(* Logix 5000 AddOnInstructionDefinition export PRNG; software revision 30.00; part 2 of 3 *)

ADD_ON_INSTRUCTION L_ADD   (* revision 1.0 00 Release, vendor Rockwell Automation *)
// Add (64-bit)
// Revision note:
// Initial Release
// Help:
// Adds two LINT (signed 64-bit) values and returns a LINT (signed 64-bit) sum.
// Also provides math status bits for Carry, Negative, Overflow and Zero result
// (equivalent to built-in S:C, S:N, S:V, S:Z).
VAR_IN_OUT
   Inp_A : LINT; {required}   // First Addend, 64-bit Integer
   Inp_B : LINT; {required}   // Second Addend, 64-bit Integer
   Out : LINT; {required}   // Sum, 64-bit Integer
END_VAR
VAR_OUTPUT
   Sts_C : BOOL; {access Read Only, visible}   // Carry result
   Sts_N : BOOL; {access Read Only, visible}   // Negative result
   Sts_V : BOOL; {access Read Only, visible}   // Overflow result
   Sts_Z : BOOL; {access Read Only, visible}   // Zero result
END_VAR
VAR
   Wrk_Sum : DINT[3];   // 20- and 24-bit fields of Out (sum)
   Wrk_B : DINT[3];   // 20- and 24-bit fields of Inp_B
   Wrk_A : DINT[3];   // 20- and 24-bit fields of Inp_A
   Wrk_Out : DINT[2];   // Output as two 32-bit DINTs
   Wrk_InpB : DINT[2];   // Input B as two 32-bit DINTs
   Wrk_InpA : DINT[2];   // Input A as two 32-bit DINTs
END_VAR

ROUTINE Logic   (* ladder *)
// Do 64-bit addition
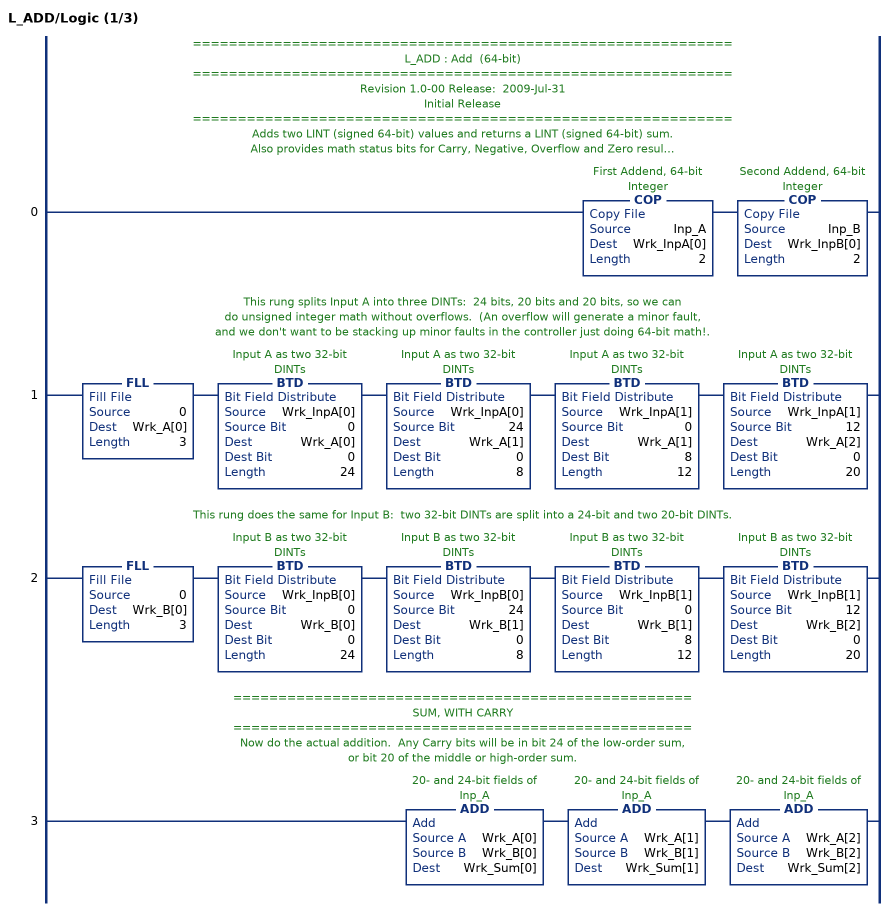
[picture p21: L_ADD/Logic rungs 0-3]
   // ============================================================
   // L_ADD : Add  (64-bit)
   // ============================================================
   // Revision 1.0-00 Release:  2009-Jul-31
   // Initial Release
   // ============================================================
   // Adds two LINT (signed 64-bit) values and returns a LINT (signed 64-bit) sum.
   // Also provides math status bits for Carry, Negative, Overflow and Zero result
   // (equivalent to built-in S:C, S:N, S:V, S:Z).
   // This instruction breaks the LINT addends into three DINTs
   // (24 bits, 20 bits and 20 bits) to do the math in order to
   // avoid generating a Controller MINOR FAULT on overflow.
   // (Sample code provided in RSLogix 5000 Online Help is much
   // smaller and faster, but causes numerous Minor Faults on
   // Overflows -- S:V -- on the low-order sum!  The controller must
   // take time to log the minor faults, and many users do not want to see
   // Minor Faults on normal math operations.  See the RSLogix 5000
   // Help Topic "Arithmetic Status Flags" for more information.)
   // ===================================================
   // CONVERT LINTs TO DINTs
   // ===================================================
   // These COPies take the input LINTs and break them into pairs of DINTs so we can do math on them.
   // Logix V17 has a LINT data type, but math instructions (and AOI Input and Output Parameters) don't support LINT.
   0: COP(Inp_A,Wrk_InpA[0],2)COP(Inp_B,Wrk_InpB[0],2);
   // This rung splits Input A into three DINTs:  24 bits, 20 bits and 20 bits, so we can
   // do unsigned integer math without overflows.  (An overflow will generate a minor fault,
   // and we don't want to be stacking up minor faults in the controller just doing 64-bit math!.
   1: FLL(0,Wrk_A[0],3)BTD(Wrk_InpA[0],0,Wrk_A[0],0,24)BTD(Wrk_InpA[0],24,Wrk_A[1],0,8)BTD(Wrk_InpA[1],0,Wrk_A[1],8,12)BTD(Wrk_InpA[1],12,Wrk_A[2],0,20);
   // This rung does the same for Input B:  two 32-bit DINTs are split into a 24-bit and two 20-bit DINTs.
   2: FLL(0,Wrk_B[0],3)BTD(Wrk_InpB[0],0,Wrk_B[0],0,24)BTD(Wrk_InpB[0],24,Wrk_B[1],0,8)BTD(Wrk_InpB[1],0,Wrk_B[1],8,12)BTD(Wrk_InpB[1],12,Wrk_B[2],0,20);
   // ===================================================
   // SUM, WITH CARRY
   // ===================================================
   // Now do the actual addition.  Any Carry bits will be in bit 24 of the low-order sum,
   // or bit 20 of the middle or high-order sum.
   3: ADD(Wrk_A[0],Wrk_B[0],Wrk_Sum[0])ADD(Wrk_A[1],Wrk_B[1],Wrk_Sum[1])ADD(Wrk_A[2],Wrk_B[2],Wrk_Sum[2]);
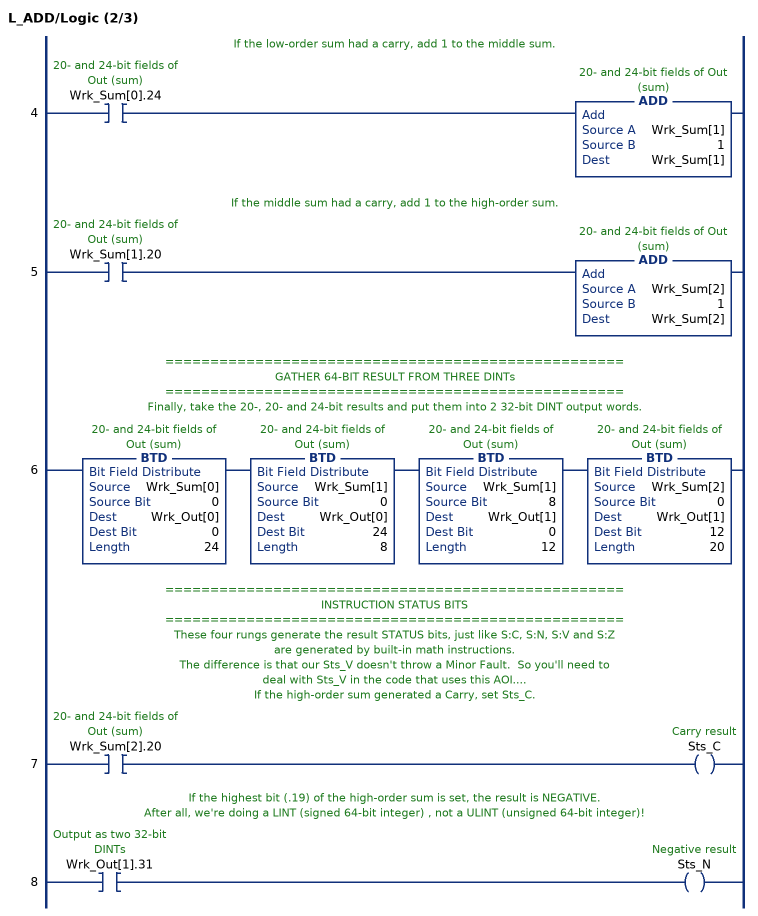
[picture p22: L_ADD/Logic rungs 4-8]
   // If the low-order sum had a carry, add 1 to the middle sum.
   4: XIC(Wrk_Sum[0].24)ADD(Wrk_Sum[1],1,Wrk_Sum[1]);
   // If the middle sum had a carry, add 1 to the high-order sum.
   5: XIC(Wrk_Sum[1].20)ADD(Wrk_Sum[2],1,Wrk_Sum[2]);
   // ===================================================
   // GATHER 64-BIT RESULT FROM THREE DINTs
   // ===================================================
   // Finally, take the 20-, 20- and 24-bit results and put them into 2 32-bit DINT output words.
   6: BTD(Wrk_Sum[0],0,Wrk_Out[0],0,24)BTD(Wrk_Sum[1],0,Wrk_Out[0],24,8)BTD(Wrk_Sum[1],8,Wrk_Out[1],0,12)BTD(Wrk_Sum[2],0,Wrk_Out[1],12,20);
   // ===================================================
   // INSTRUCTION STATUS BITS
   // ===================================================
   // These four rungs generate the result STATUS bits, just like S:C, S:N, S:V and S:Z
   // are generated by built-in math instructions.
   // The difference is that our Sts_V doesn't throw a Minor Fault.  So you'll need to
   // deal with Sts_V in the code that uses this AOI....
   // If the high-order sum generated a Carry, set Sts_C.
   7: XIC(Wrk_Sum[2].20)OTE(Sts_C);
   // If the highest bit (.19) of the high-order sum is set, the result is NEGATIVE.
   // After all, we're doing a LINT (signed 64-bit integer) , not a ULINT (unsigned 64-bit integer)!
   8: XIC(Wrk_Out[1].31)OTE(Sts_N);
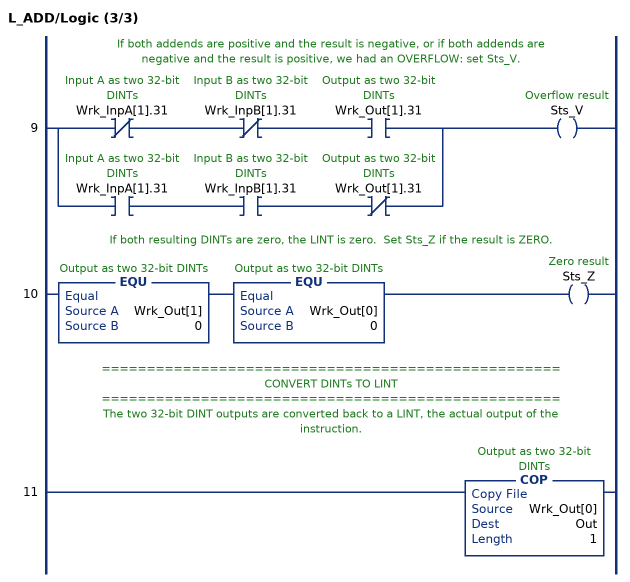
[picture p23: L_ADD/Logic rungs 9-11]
   // If both addends are positive and the result is negative, or if both addends are
   // negative and the result is positive, we had an OVERFLOW: set Sts_V.
   9: [XIO(Wrk_InpA[1].31) XIO(Wrk_InpB[1].31) XIC(Wrk_Out[1].31) ,XIC(Wrk_InpA[1].31) XIC(Wrk_InpB[1].31) XIO(Wrk_Out[1].31) ]OTE(Sts_V);
   // If both resulting DINTs are zero, the LINT is zero.  Set Sts_Z if the result is ZERO.
   10: EQU(Wrk_Out[1],0)EQU(Wrk_Out[0],0)OTE(Sts_Z);
   // ===================================================
   // CONVERT DINTs TO LINT
   // ===================================================
   // The two 32-bit DINT outputs are converted back to a LINT, the actual output of the instruction.
   11: COP(Wrk_Out[0],Out,1);
END_ROUTINE
END_ADD_ON_INSTRUCTION

ADD_ON_INSTRUCTION L_AND   (* revision 1.0 00 Release, vendor Rockwell Automation *)
// Bitwise AND (64-bit)
// Revision note:
// Initial Release
// Help:
// This instruction returns the bitwise Logical AND (output bit true if both corresponding
// input bits true) of two input 64-bit integers (LINTs), into an output 64-bit integer.
VAR_IN_OUT
   Inp_A : LINT; {required}   // Input A
   Inp_B : LINT; {required}   // Input B
   Out : LINT; {required}   // Output = Input A & Input B
END_VAR
VAR
   Wrk_Out : DINT[2];   // Output as two 32-bit DINTs
   Wrk_InpB : DINT[2];   // Input B as two 32-bit DINTs
   Wrk_InpA : DINT[2];   // Input A as two 32-bit DINTs
END_VAR

ROUTINE Logic   (* ladder *)
// Perform 64-bit bitwise logical AND
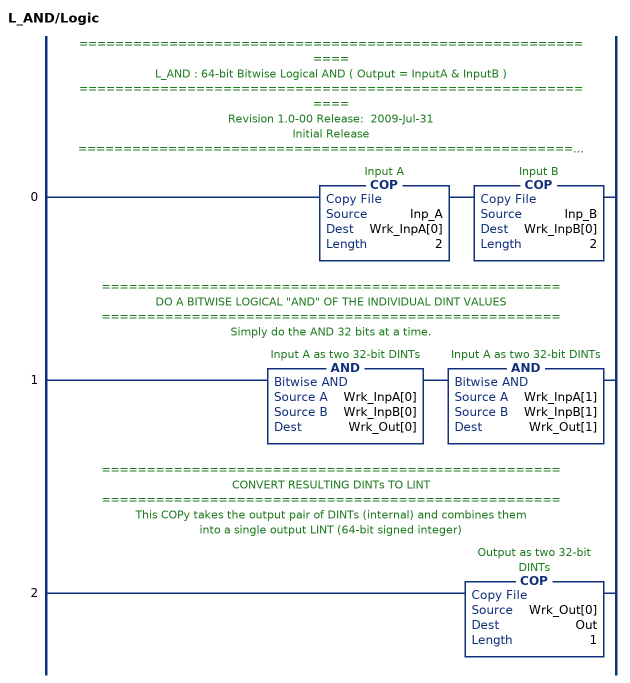
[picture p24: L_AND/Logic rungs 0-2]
   // ============================================================
   // L_AND : 64-bit Bitwise Logical AND ( Output = InputA & InputB )
   // ============================================================
   // Revision 1.0-00 Release:  2009-Jul-31
   // Initial Release
   // ============================================================
   // Returns the bitwise Logical AND of the input 64-bit integer (LINT) values.
   // This rung breaks each LINT input into two DINTs
   // (32-bit signed each) to do the logical AND function.
   // ===================================================
   // CONVERT LINTs TO DINTs
   // ===================================================
   // These COPies take the input LINT values and break them into a pair of DINTs each.
   0: COP(Inp_A,Wrk_InpA[0],2)COP(Inp_B,Wrk_InpB[0],2);
   // ===================================================
   // DO A BITWISE LOGICAL "AND" OF THE INDIVIDUAL DINT VALUES
   // ===================================================
   // Simply do the AND 32 bits at a time.
   1: AND(Wrk_InpA[0],Wrk_InpB[0],Wrk_Out[0])AND(Wrk_InpA[1],Wrk_InpB[1],Wrk_Out[1]);
   // ===================================================
   // CONVERT RESULTING DINTs TO LINT
   // ===================================================
   // This COPy takes the output pair of DINTs (internal) and combines them
   // into a single output LINT (64-bit signed integer)
   2: COP(Wrk_Out[0],Out,1);
END_ROUTINE
END_ADD_ON_INSTRUCTION

ADD_ON_INSTRUCTION L_NOT   (* revision 1.0 00 Release, vendor Rockwell Automation *)
// Bitwise NOT (64-bit)
// Revision note:
// Initial Release
// Help:
// This instruction returns the bitwise Logical NOT (inverse or 1's complement)
// of an input 64-bit integer (LINT) value.  (It flips all the bits.)
VAR_IN_OUT
   Inp : LINT; {required}   // Input
   Out : LINT; {required}   // Output = - Input
END_VAR
VAR
   Wrk : DINT[2];   // 32-bit portions of Input
END_VAR

ROUTINE Logic   (* ladder *)
// Perform a bitwise logical NOT (invert)
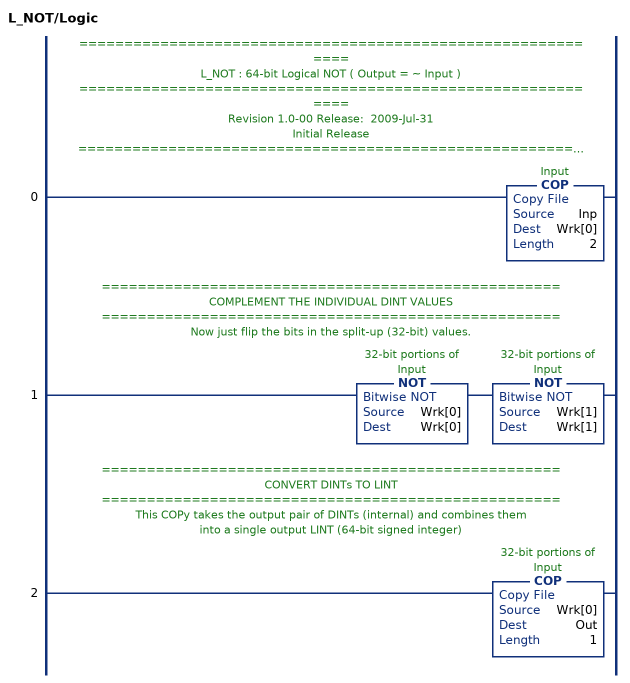
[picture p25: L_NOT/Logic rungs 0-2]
   // ============================================================
   // L_NOT : 64-bit Logical NOT ( Output = ~ Input )
   // ============================================================
   // Revision 1.0-00 Release:  2009-Jul-31
   // Initial Release
   // ============================================================
   // Returns the Logical NOT (1's complement, all bits flipped)
   // of the input 64-bit integer (LINT) value.
   // This instruction breaks the LINT input into two DINTs
   // (32-bit signed each) to do the inverting.
   // ===================================================
   // CONVERT LINT TO DINTs
   // ===================================================
   // This COPy takes the input LINT and breaks it into a pair of DINTs.
   0: COP(Inp,Wrk[0],2);
   // ===================================================
   // COMPLEMENT THE INDIVIDUAL DINT VALUES
   // ===================================================
   // Now just flip the bits in the split-up (32-bit) values.
   1: NOT(Wrk[0],Wrk[0])NOT(Wrk[1],Wrk[1]);
   // ===================================================
   // CONVERT DINTs TO LINT
   // ===================================================
   // This COPy takes the output pair of DINTs (internal) and combines them
   // into a single output LINT (64-bit signed integer)
   2: COP(Wrk[0],Out,1);
END_ROUTINE
END_ADD_ON_INSTRUCTION

ADD_ON_INSTRUCTION L_ROTR   (* revision 1.0 20170524, vendor Kenneth A. Fischer *)
// LINT circular right shift (rotation) of the 64-bit argument Inp_A by Inp_B bits
// Revision note:
// Rev1.0: 20170524 - Initial Release
VAR_IN_OUT
   Inp_A : LINT; {required}   // 64-bit Integer to be right circular rotated
END_VAR
VAR_INPUT
   Inp_B : INT; {required}   // Number of Inp_A bit rotations
END_VAR
VAR_IN_OUT
   Out : LINT; {required}   // Result
END_VAR
VAR
   Wrk_InpA : DINT[2];   // Input A as two 32-bit DINTs
   BSR_Cntrl : CONTROL := (LEN := 64);
   Source_Bit : BOOL;
   ONS : BOOL;
END_VAR

ROUTINE Logic   (* ladder *)
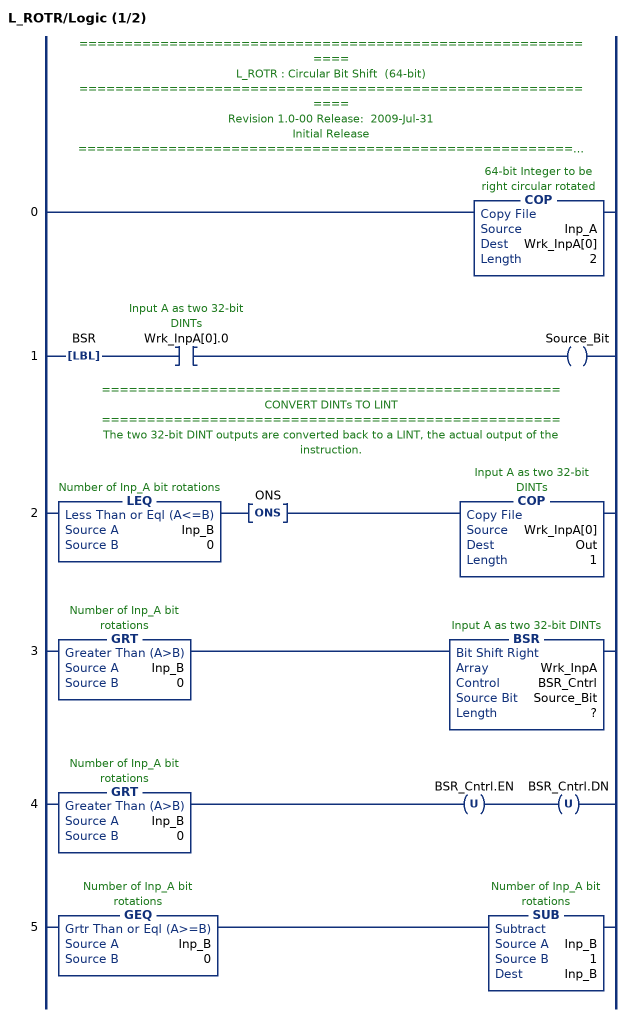
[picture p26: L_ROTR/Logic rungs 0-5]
   // ============================================================
   // L_ROTR : Circular Bit Shift  (64-bit)
   // ============================================================
   // Revision 1.0-00 Release:  2009-Jul-31
   // Initial Release
   // ============================================================
   // Performs a circular right shift rotation of the 64-bit argument Inp_A by the
   // number of bits defined in the 16-bit argument Inp_B.
   // ===================================================
   // CONVERT LINTs TO DINTs
   // ===================================================
   // These COPies take the input LINTs and break them into pairs of DINTs so we can do math on them.
   // Logix V17 has a LINT data type, but math instructions (and AOI Input and Output Parameters) don't support LINT.
   0: COP(Inp_A,Wrk_InpA[0],2);
   1: LBL(BSR)XIC(Wrk_InpA[0].0)OTE(Source_Bit);
   // ===================================================
   // CONVERT DINTs TO LINT
   // ===================================================
   // The two 32-bit DINT outputs are converted back to a LINT, the actual output of the instruction.
   2: LEQ(Inp_B,0)ONS(ONS)COP(Wrk_InpA[0],Out,1);
   3: GRT(Inp_B,0)BSR(Wrk_InpA,BSR_Cntrl,Source_Bit,?);
   4: GRT(Inp_B,0)OTU(BSR_Cntrl.EN)OTU(BSR_Cntrl.DN);
   5: GEQ(Inp_B,0)SUB(Inp_B,1,Inp_B);
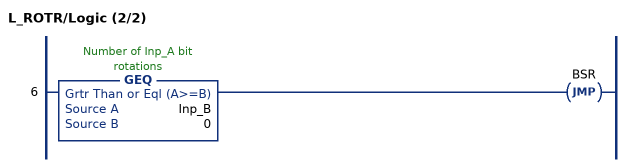
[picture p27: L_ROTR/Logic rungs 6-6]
   6: GEQ(Inp_B,0)JMP(BSR);
END_ROUTINE
END_ADD_ON_INSTRUCTION

ADD_ON_INSTRUCTION L_SHR   (* revision 1.0 20170524, vendor Kenneth A. Fischer *)
// LINT bit shift right of the 64-bit argument Inp_A by Inp_B bits with paddding by zeros on the right
// Revision note:
// Rev1.0: 20170524 - Initial Release
VAR_IN_OUT
   Inp_A : LINT; {required}   // 64-bit Integer to be right circular rotated
END_VAR
VAR_INPUT
   Inp_B : INT; {required}   // Number of bits to shift
END_VAR
VAR_IN_OUT
   Out : LINT; {required}   // Result
END_VAR
VAR
   BSR_Cntrl : CONTROL := (LEN := 64);
   ONS : BOOL;
   Source_Bit : BOOL;
   Wrk_InpA : DINT[2];   // Input A as two 32-bit DINTs
END_VAR

ROUTINE Logic   (* ladder *)
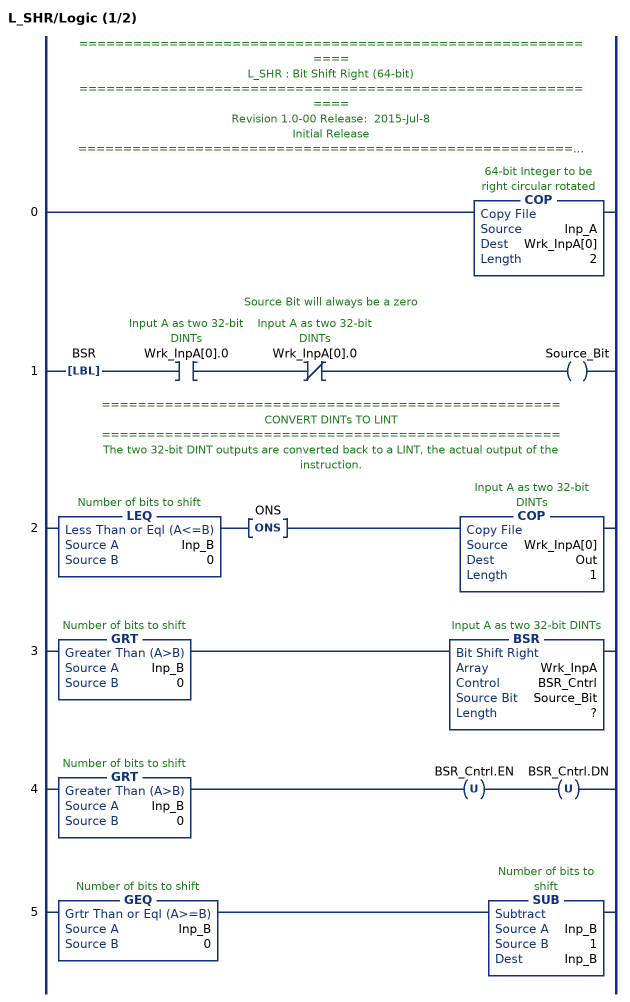
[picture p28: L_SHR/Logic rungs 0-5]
   // ============================================================
   // L_SHR : Bit Shift Right (64-bit)
   // ============================================================
   // Revision 1.0-00 Release:  2015-Jul-8
   // Initial Release
   // ============================================================
   // Performs a right bit shift of the 64-bit argument Inp_A by the
   // number of bits defined in the 16-bit argument Inp_B, with padding by zeros.
   // ===================================================
   // CONVERT LINTs TO DINTs
   // ===================================================
   // These COPies take the input LINTs and break them into pairs of DINTs so we can do math on them.
   // Logix V17 has a LINT data type, but math instructions (and AOI Input and Output Parameters) don't support LINT.
   0: COP(Inp_A,Wrk_InpA[0],2);
   // Source Bit will always be a zero
   1: LBL(BSR)XIC(Wrk_InpA[0].0)XIO(Wrk_InpA[0].0)OTE(Source_Bit);
   // ===================================================
   // CONVERT DINTs TO LINT
   // ===================================================
   // The two 32-bit DINT outputs are converted back to a LINT, the actual output of the instruction.
   2: LEQ(Inp_B,0)ONS(ONS)COP(Wrk_InpA[0],Out,1);
   3: GRT(Inp_B,0)BSR(Wrk_InpA,BSR_Cntrl,Source_Bit,?);
   4: GRT(Inp_B,0)OTU(BSR_Cntrl.EN)OTU(BSR_Cntrl.DN);
   5: GEQ(Inp_B,0)SUB(Inp_B,1,Inp_B);
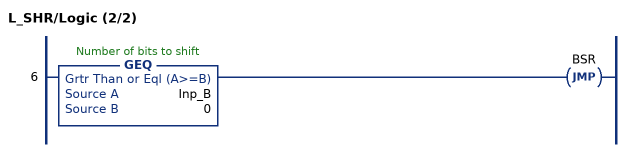
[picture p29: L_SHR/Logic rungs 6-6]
   6: GEQ(Inp_B,0)JMP(BSR);
END_ROUTINE
END_ADD_ON_INSTRUCTION

ADD_ON_INSTRUCTION L_XOR   (* revision 1.0 00 Release, vendor Rockwell Automation *)
// Bitwise XOR (64-bit)
// Revision note:
// Initial Release
// Help:
// This instruction returns the bitwise Logical XOR (exclusive OR, output
// bit true if either but NOT both of the corresponding input bits are true)
// of two input 64-bit integers (LINTs), into an output 64-bit integer.
VAR_IN_OUT
   Inp_A : LINT; {required}   // Input A
   Inp_B : LINT; {required}   // Input B
   Out : LINT; {required}   // Output = Input A | Input B
END_VAR
VAR
   Wrk_Out : DINT[2];   // Output as two 32-bit DINTs
   Wrk_InpB : DINT[2];   // Input B as two 32-bit DINTs
   Wrk_InpA : DINT[2];   // Input A as two 32-bit DINTs
END_VAR

ROUTINE Logic   (* ladder *)
// Perform bitwise logical XOR
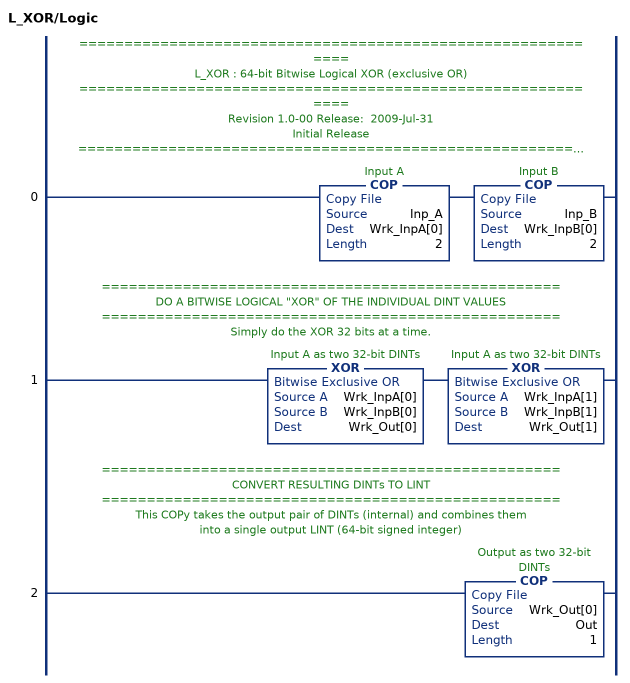
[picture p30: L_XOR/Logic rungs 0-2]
   // ============================================================
   // L_XOR : 64-bit Bitwise Logical XOR (exclusive OR)
   // ============================================================
   // Revision 1.0-00 Release:  2009-Jul-31
   // Initial Release
   // ============================================================
   // Returns the bitwise Logical XOR of the input 64-bit integer (LINT) values.
   // This rung breaks each LINT input into two DINTs
   // (32-bit signed each) to do the logical XOR function.
   // ===================================================
   // CONVERT LINTs TO DINTs
   // ===================================================
   // These COPies take the input LINT values and break them into a pair of DINTs each.
   0: COP(Inp_A,Wrk_InpA[0],2)COP(Inp_B,Wrk_InpB[0],2);
   // ===================================================
   // DO A BITWISE LOGICAL "XOR" OF THE INDIVIDUAL DINT VALUES
   // ===================================================
   // Simply do the XOR 32 bits at a time.
   1: XOR(Wrk_InpA[0],Wrk_InpB[0],Wrk_Out[0])XOR(Wrk_InpA[1],Wrk_InpB[1],Wrk_Out[1]);
   // ===================================================
   // CONVERT RESULTING DINTs TO LINT
   // ===================================================
   // This COPy takes the output pair of DINTs (internal) and combines them
   // into a single output LINT (64-bit signed integer)
   2: COP(Wrk_Out[0],Out,1);
END_ROUTINE
END_ADD_ON_INSTRUCTION

ADD_ON_INSTRUCTION SHA512_SEQ   (* revision 1.0 20170916, vendor Kenneth A. Fischer *)
// Generates SHA 512 hash of data.
// Revision note:
// Rev1.0: 20170916 - Initial Release
VAR_IN_OUT
   Inp_MSG : LINT[1600]; {required}
END_VAR
VAR_INPUT
   Inp_LEN : DINT; {required}   // LENGTH INPUT OF MSG IN NUMBER OF LINTS
END_VAR
VAR_IN_OUT
   Out_HASH : LINT[8]; {required}
        [0]   // HashBuffer_A
        [1]   // HashBuffer_B
        [2]   // HashBuffer_C
        [3]   // HashBuffer_D
        [4]   // HashBuffer_E
        [5]   // HashBuffer_F
        [6]   // HashBuffer_G
        [7]   // HashBuffer_H
END_VAR
VAR_OUTPUT
   SEQCTRL_DN : BOOL; {access Read Only}   // Complete
END_VAR
VAR_INPUT
   SEQCTRL_RESET : BOOL;   // Resets Point Multiplication if Toggled True
END_VAR
VAR_OUTPUT
   SEQCTRL_STEP : INT; {access Read Only}
END_VAR
VAR
   SEQCTRL_CMD : DINT;
   SEQCTRL_CMD_TABLE : DINT[100];
   SEQCTRL_DONE : DINT;
   SEQCTRL_NEXT_STEP : INT;
   i : INT;
   ALWAYS_OFF : BOOL;
   CondFunc : LINT;
   CondFunc_tmp : LINT[3];
   HashBuffer_A : LINT;
   HashBuffer_B : LINT;
   HashBuffer_C : LINT;
   HashBuffer_D : LINT;
   HashBuffer_E : LINT;
   HashBuffer_F : LINT;
   HashBuffer_G : LINT;
   HashBuffer_H : LINT;
   HashBufferInput_A : LINT;
   HashBufferInput_B : LINT;
   HashBufferInput_C : LINT;
   HashBufferInput_D : LINT;
   HashBufferInput_E : LINT;
   HashBufferInput_F : LINT;
   HashBufferInput_G : LINT;
   HashBufferInput_H : LINT;
   M : INT;   // MESSAGE INCREMENTS
   t : INT;
   K : LINT[85];
   L_ADD : L_ADD;
   L_ADD1 : L_ADD;
   L_AND : L_AND;
   L_NOT : L_NOT;
   L_ROTR : L_ROTR;
   L_SHR : L_SHR;
   L_XOR : L_XOR;
   LENGTH_BITS : DINT;   // LENGTH OF MSG IN BITS
   LENGTH_MODULO : DINT;
   MajFunc : LINT;
   NUM_PADDING_BITS : DINT;   // NUMBER OF BITS NEEDED FOR PADDING
   NUM_PADDING_LINTS : DINT;   // NUMBER OF LINTS NEEDED FOR PADDING
   PADDING_COUNTER : DINT;
   Sigma0 : LINT;
   Sigma1 : LINT;
   SigmaA : LINT;
   SigmaE : LINT;
   x : INT;
   j : INT;
   T1 : LINT;
   T2 : LINT;
   tmp : LINT[20];
   tmp1 : DINT;
   tmp2 : DINT;
   TOTAL_MSG_LENGTH_MINUS_16 : DINT;
   W : LINT[85];   // MESSAGE SCHEDULE
   Wrk : DINT[2];
   TEMP : DINT;
END_VAR

ROUTINE Logic   (* ladder *)
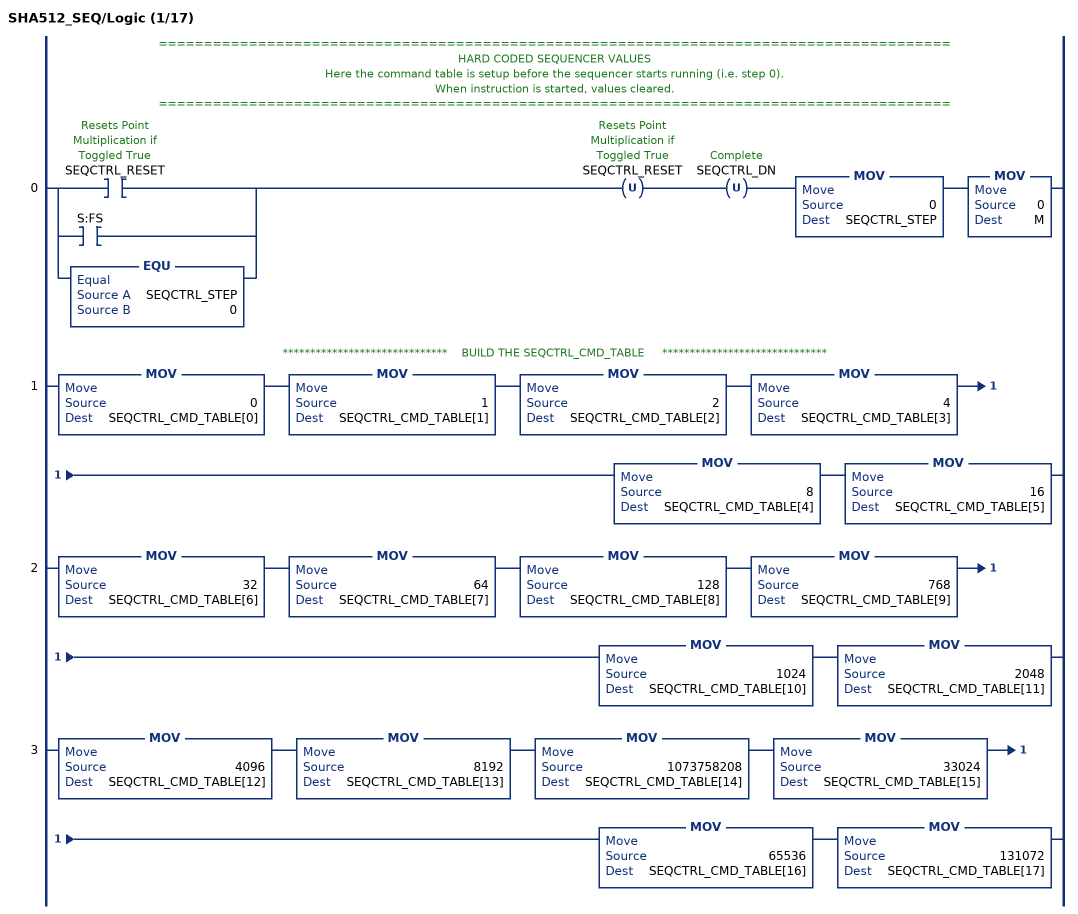
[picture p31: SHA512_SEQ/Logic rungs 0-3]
   // ========================================================================================
   // HARD CODED SEQUENCER VALUES
   // Here the command table is setup before the sequencer starts running (i.e. step 0).
   // When instruction is started, values cleared.
   // ========================================================================================
   0: [[XIC(SEQCTRL_RESET) ,XIC(S:FS) ] ,EQU(SEQCTRL_STEP,0) ]OTU(SEQCTRL_RESET)OTU(SEQCTRL_DN)MOV(0,SEQCTRL_STEP)MOV(0,M);
   // ******************************    BUILD THE SEQCTRL_CMD_TABLE     ******************************
   1: MOV(0,SEQCTRL_CMD_TABLE[0])MOV(1,SEQCTRL_CMD_TABLE[1])MOV(2,SEQCTRL_CMD_TABLE[2])MOV(4,SEQCTRL_CMD_TABLE[3])MOV(8,SEQCTRL_CMD_TABLE[4])MOV(16,SEQCTRL_CMD_TABLE[5]);
   2: MOV(32,SEQCTRL_CMD_TABLE[6])MOV(64,SEQCTRL_CMD_TABLE[7])MOV(128,SEQCTRL_CMD_TABLE[8])MOV(768,SEQCTRL_CMD_TABLE[9])MOV(1024,SEQCTRL_CMD_TABLE[10])MOV(2048,SEQCTRL_CMD_TABLE[11]);
   3: MOV(4096,SEQCTRL_CMD_TABLE[12])MOV(8192,SEQCTRL_CMD_TABLE[13])MOV(1073758208,SEQCTRL_CMD_TABLE[14])MOV(33024,SEQCTRL_CMD_TABLE[15])MOV(65536,SEQCTRL_CMD_TABLE[16])MOV(131072,SEQCTRL_CMD_TABLE[17]);
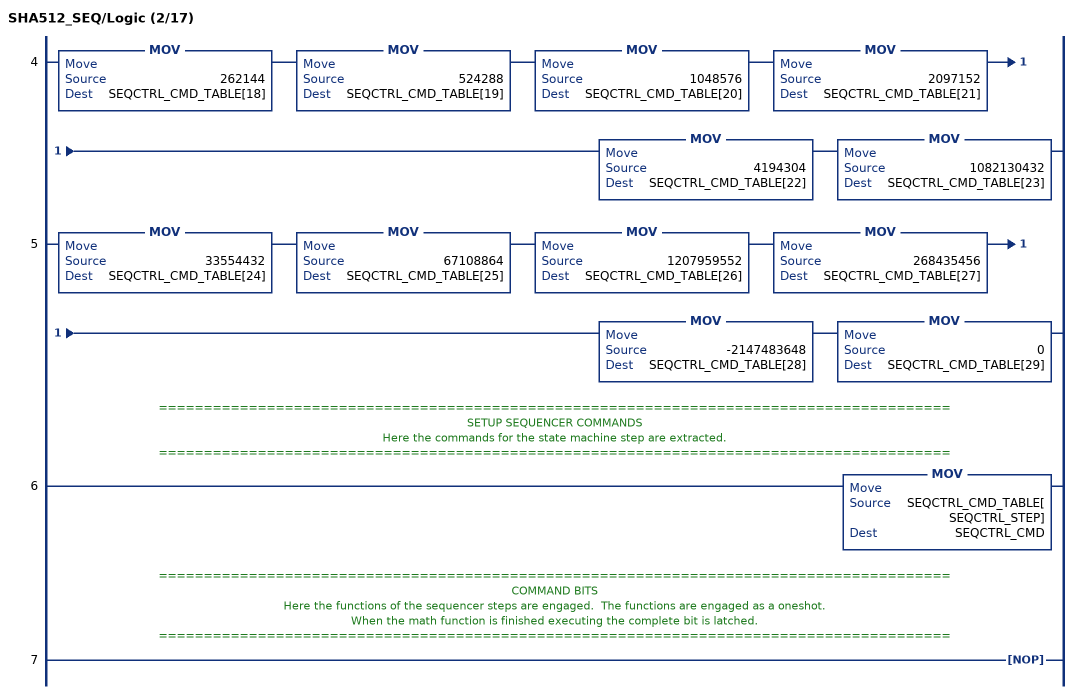
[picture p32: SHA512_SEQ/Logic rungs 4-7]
   4: MOV(262144,SEQCTRL_CMD_TABLE[18])MOV(524288,SEQCTRL_CMD_TABLE[19])MOV(1048576,SEQCTRL_CMD_TABLE[20])MOV(2097152,SEQCTRL_CMD_TABLE[21])MOV(4194304,SEQCTRL_CMD_TABLE[22])MOV(1082130432,SEQCTRL_CMD_TABLE[23]);
   5: MOV(33554432,SEQCTRL_CMD_TABLE[24])MOV(67108864,SEQCTRL_CMD_TABLE[25])MOV(1207959552,SEQCTRL_CMD_TABLE[26])MOV(268435456,SEQCTRL_CMD_TABLE[27])MOV(-2147483648,SEQCTRL_CMD_TABLE[28])MOV(0,SEQCTRL_CMD_TABLE[29]);
   // ========================================================================================
   // SETUP SEQUENCER COMMANDS
   // Here the commands for the state machine step are extracted.
   // ========================================================================================
   6: MOV(SEQCTRL_CMD_TABLE[SEQCTRL_STEP],SEQCTRL_CMD);
   // ========================================================================================
   // COMMAND BITS
   // Here the functions of the sequencer steps are engaged.  The functions are engaged as a oneshot.
   // When the math function is finished executing the complete bit is latched.
   // ========================================================================================
   7: NOP();
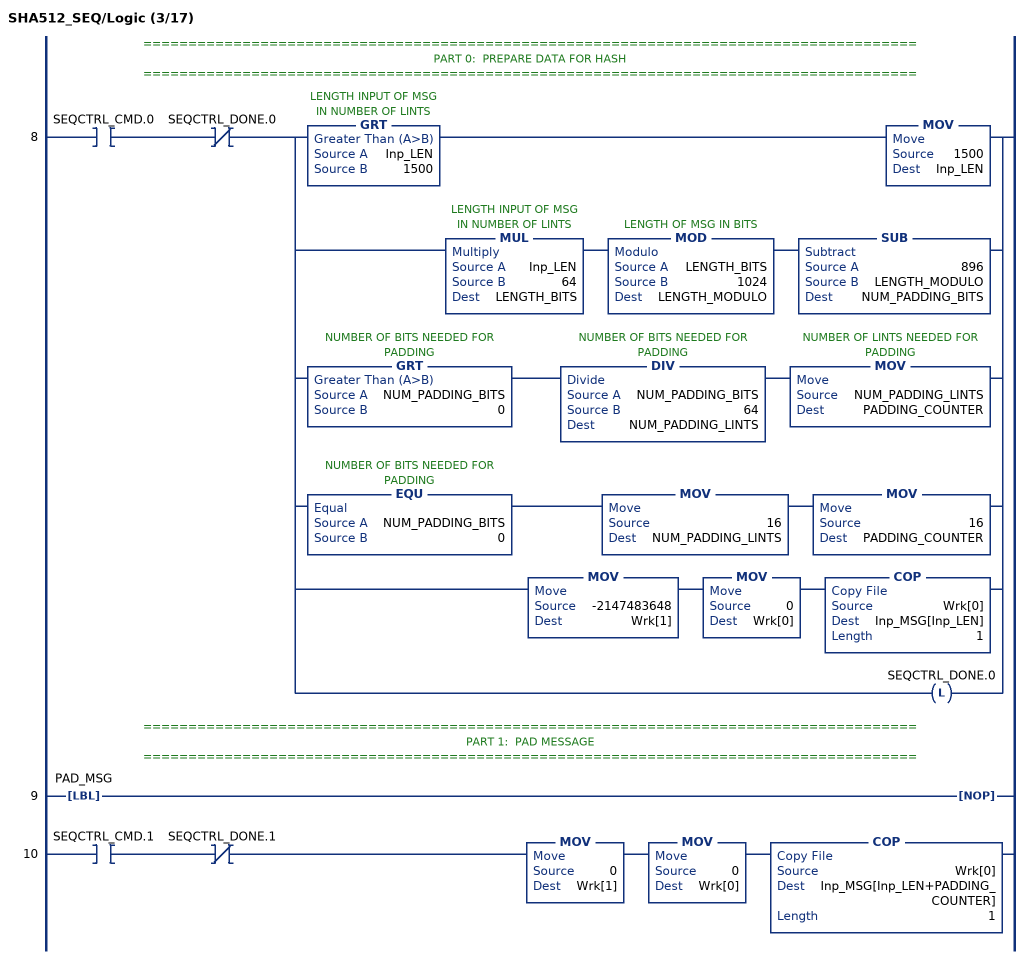
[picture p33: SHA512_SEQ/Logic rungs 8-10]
   // ======================================================================================
   // PART 0:  PREPARE DATA FOR HASH
   // ======================================================================================
   8: XIC(SEQCTRL_CMD.0)XIO(SEQCTRL_DONE.0)[GRT(Inp_LEN,1500) MOV(1500,Inp_LEN) ,MUL(Inp_LEN,64,LENGTH_BITS) MOD(LENGTH_BITS,1024,LENGTH_MODULO) SUB(896,LENGTH_MODULO,NUM_PADDING_BITS) ,GRT(NUM_PADDING_BITS,0) DIV(NUM_PADDING_BITS,64,NUM_PADDING_LINTS) MOV(NUM_PADDING_LINTS,PADDING_COUNTER) ,EQU(NUM_PADDING_BITS,0) MOV(16,NUM_PADDING_LINTS) MOV(16,PADDING_COUNTER) ,MOV(-2147483648,Wrk[1]) MOV(0,Wrk[0]) COP(Wrk[0],Inp_MSG[Inp_LEN],1) ,OTL(SEQCTRL_DONE.0) ];
   // ======================================================================================
   // PART 1:  PAD MESSAGE
   // ======================================================================================
   9: LBL(PAD_MSG)NOP();
   10: XIC(SEQCTRL_CMD.1)XIO(SEQCTRL_DONE.1)MOV(0,Wrk[1])MOV(0,Wrk[0])COP(Wrk[0],Inp_MSG[Inp_LEN+PADDING_COUNTER],1);
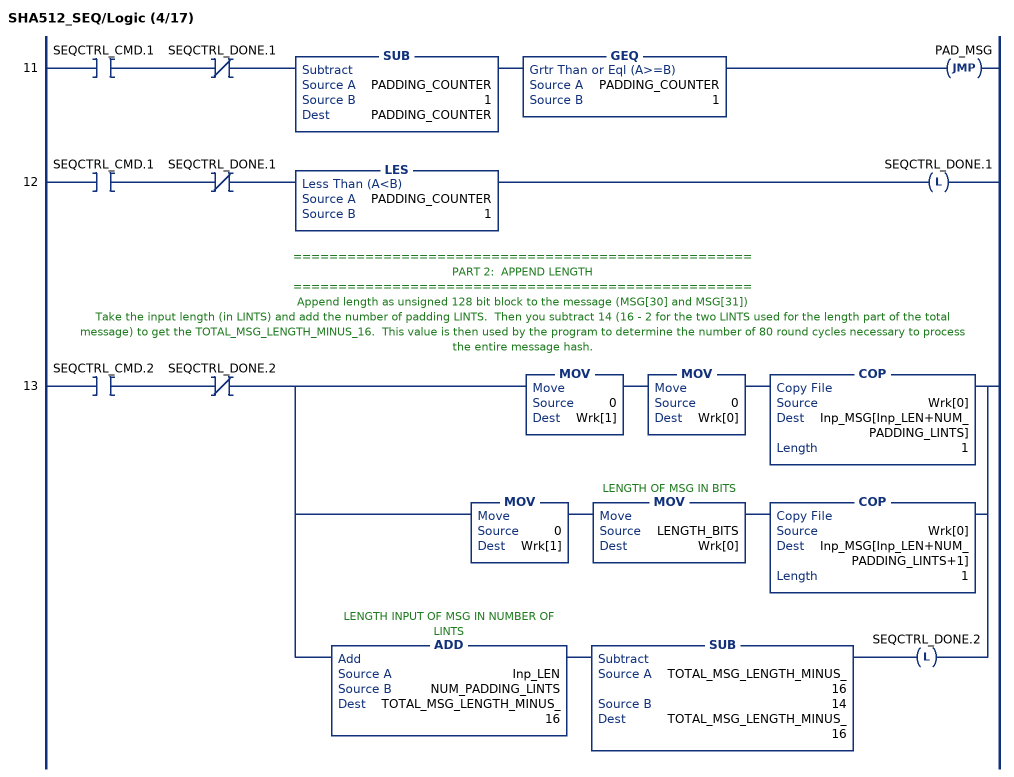
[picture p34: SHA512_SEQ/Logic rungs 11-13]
   11: XIC(SEQCTRL_CMD.1)XIO(SEQCTRL_DONE.1)SUB(PADDING_COUNTER,1,PADDING_COUNTER)GEQ(PADDING_COUNTER,1)JMP(PAD_MSG);
   12: XIC(SEQCTRL_CMD.1)XIO(SEQCTRL_DONE.1)LES(PADDING_COUNTER,1)OTL(SEQCTRL_DONE.1);
   // ===================================================
   // PART 2:  APPEND LENGTH
   // ===================================================
   // Append length as unsigned 128 bit block to the message (MSG[30] and MSG[31])
   // Take the input length (in LINTS) and add the number of padding LINTS.  Then you subtract 14 (16 - 2 for the two LINTS used for the length part of the total message) to get the TOTAL_MSG_LENGTH_MINUS_16.  This value is then used by the program to determine the number of 80 round cycles necessary to process the entire message hash.
   13: XIC(SEQCTRL_CMD.2)XIO(SEQCTRL_DONE.2)[MOV(0,Wrk[1]) MOV(0,Wrk[0]) COP(Wrk[0],Inp_MSG[Inp_LEN+NUM_PADDING_LINTS],1) ,MOV(0,Wrk[1]) MOV(LENGTH_BITS,Wrk[0]) COP(Wrk[0],Inp_MSG[Inp_LEN+NUM_PADDING_LINTS+1],1) ,ADD(Inp_LEN,NUM_PADDING_LINTS,TOTAL_MSG_LENGTH_MINUS_16) SUB(TOTAL_MSG_LENGTH_MINUS_16,14,TOTAL_MSG_LENGTH_MINUS_16) OTL(SEQCTRL_DONE.2) ];
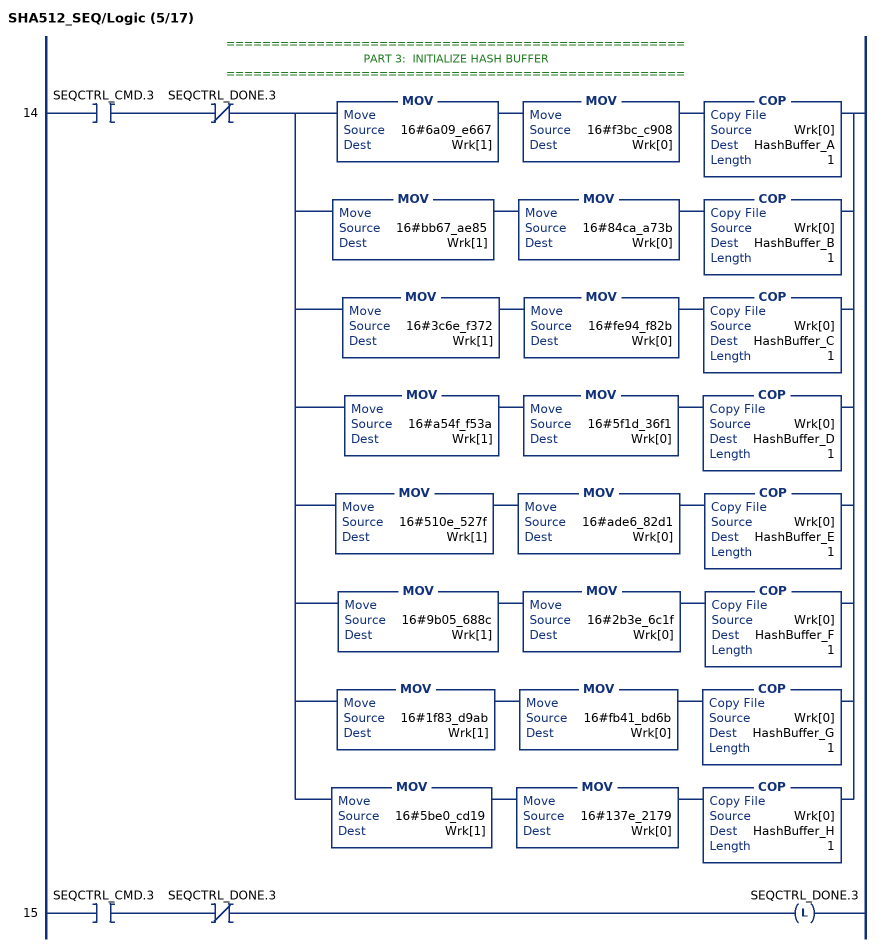
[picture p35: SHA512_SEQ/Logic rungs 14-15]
   // ===================================================
   // PART 3:  INITIALIZE HASH BUFFER
   // ===================================================
   14: XIC(SEQCTRL_CMD.3)XIO(SEQCTRL_DONE.3)[MOV(16#6a09_e667,Wrk[1]) MOV(16#f3bc_c908,Wrk[0]) COP(Wrk[0],HashBuffer_A,1) ,MOV(16#bb67_ae85,Wrk[1]) MOV(16#84ca_a73b,Wrk[0]) COP(Wrk[0],HashBuffer_B,1) ,MOV(16#3c6e_f372,Wrk[1]) MOV(16#fe94_f82b,Wrk[0]) COP(Wrk[0],HashBuffer_C,1) ,MOV(16#a54f_f53a,Wrk[1]) MOV(16#5f1d_36f1,Wrk[0]) COP(Wrk[0],HashBuffer_D,1) ,MOV(16#510e_527f,Wrk[1]) MOV(16#ade6_82d1,Wrk[0]) COP(Wrk[0],HashBuffer_E,1) ,MOV(16#9b05_688c,Wrk[1]) MOV(16#2b3e_6c1f,Wrk[0]) COP(Wrk[0],HashBuffer_F,1) ,MOV(16#1f83_d9ab,Wrk[1]) MOV(16#fb41_bd6b,Wrk[0]) COP(Wrk[0],HashBuffer_G,1) ,MOV(16#5be0_cd19,Wrk[1]) MOV(16#137e_2179,Wrk[0]) COP(Wrk[0],HashBuffer_H,1) ];
   15: XIC(SEQCTRL_CMD.3)XIO(SEQCTRL_DONE.3)OTL(SEQCTRL_DONE.3);
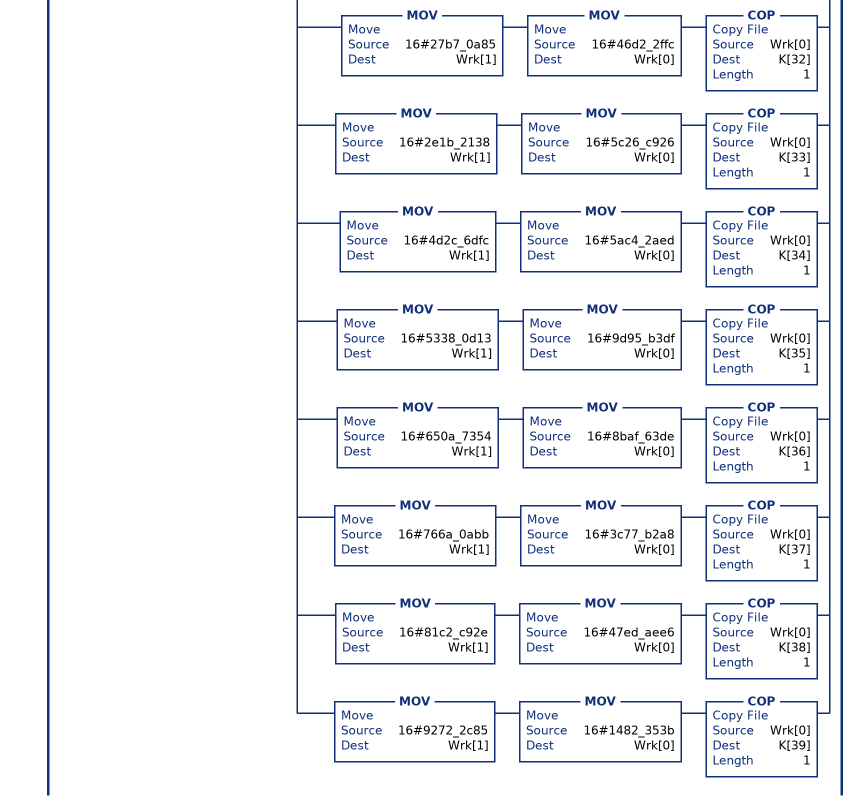
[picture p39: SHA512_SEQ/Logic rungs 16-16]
   // ===================================================
   // PART 4:  INITIALIZE K CONSTANTS - PART 1
   // ===================================================
   16: XIC(SEQCTRL_CMD.4)XIO(SEQCTRL_DONE.4)[MOV(16#428a_2f98,Wrk[1]) MOV(16#d728_ae22,Wrk[0]) COP(Wrk[0],K[0],1) ,MOV(16#7137_4491,Wrk[1]) MOV(16#23ef_65cd,Wrk[0]) COP(Wrk[0],K[1],1) ,MOV(16#b5c0_fbcf,Wrk[1]) MOV(16#ec4d_3b2f,Wrk[0]) COP(Wrk[0],K[2],1) ,MOV(16#e9b5_dba5,Wrk[1]) MOV(16#8189_dbbc,Wrk[0]) COP(Wrk[0],K[3],1) ,MOV(16#3956_c25b,Wrk[1]) MOV(16#f348_b538,Wrk[0]) COP(Wrk[0],K[4],1) ,MOV(16#59f1_11f1,Wrk[1]) MOV(16#b605_d019,Wrk[0]) COP(Wrk[0],K[5],1) ,MOV(16#923f_82a4,Wrk[1]) MOV(16#af19_4f9b,Wrk[0]) COP(Wrk[0],K[6],1) ,MOV(16#ab1c_5ed5,Wrk[1]) MOV(16#da6d_8118,Wrk[0]) COP(Wrk[0],K[7],1) ,MOV(16#d807_aa98,Wrk[1]) MOV(16#a303_0242,Wrk[0]) COP(Wrk[0],K[8],1) ,MOV(16#1283_5b01,Wrk[1]) MOV(16#4570_6fbe,Wrk[0]) COP(Wrk[0],K[9],1) ,MOV(16#2431_85be,Wrk[1]) MOV(16#4ee4_b28c,Wrk[0]) COP(Wrk[0],K[10],1) ,MOV(16#550c_7dc3,Wrk[1]) MOV(16#d5ff_b4e2,Wrk[0]) COP(Wrk[0],K[11],1) ,MOV(16#72be_5d74,Wrk[1]) MOV(16#f27b_896f,Wrk[0]) COP(Wrk[0],K[12],1) ,MOV(16#80de_b1fe,Wrk[1]) MOV(16#3b16_96b1,Wrk[0]) COP(Wrk[0],K[13],1) ,MOV(16#9bdc_06a7,Wrk[1]) MOV(16#25c7_1235,Wrk[0]) COP(Wrk[0],K[14],1) ,MOV(16#c19b_f174,Wrk[1]) MOV(16#cf69_2694,Wrk[0]) COP(Wrk[0],K[15],1) ,MOV(16#e49b_69c1,Wrk[1]) MOV(16#9ef1_4ad2,Wrk[0]) COP(Wrk[0],K[16],1) ,MOV(16#efbe_4786,Wrk[1]) MOV(16#384f_25e3,Wrk[0]) COP(Wrk[0],K[17],1) ,MOV(16#0fc1_9dc6,Wrk[1]) MOV(16#8b8c_d5b5,Wrk[0]) COP(Wrk[0],K[18],1) ,MOV(16#240c_a1cc,Wrk[1]) MOV(16#77ac_9c65,Wrk[0]) COP(Wrk[0],K[19],1) ,MOV(16#2de9_2c6f,Wrk[1]) MOV(16#592b_0275,Wrk[0]) COP(Wrk[0],K[20],1) ,MOV(16#4a74_84aa,Wrk[1]) MOV(16#6ea6_e483,Wrk[0]) COP(Wrk[0],K[21],1) ,MOV(16#5cb0_a9dc,Wrk[1]) MOV(16#bd41_fbd4,Wrk[0]) COP(Wrk[0],K[22],1) ,MOV(16#76f9_88da,Wrk[1]) MOV(16#8311_53b5,Wrk[0]) COP(Wrk[0],K[23],1) ,MOV(16#983e_5152,Wrk[1]) MOV(16#ee66_dfab,Wrk[0]) COP(Wrk[0],K[24],1) ,MOV(16#a831_c66d,Wrk[1]) MOV(16#2db4_3210,Wrk[0]) COP(Wrk[0],K[25],1) ,MOV(16#b003_27c8,Wrk[1]) MOV(16#98fb_213f,Wrk[0]) COP(Wrk[0],K[26],1) ,MOV(16#bf59_7fc7,Wrk[1]) MOV(16#beef_0ee4,Wrk[0]) COP(Wrk[0],K[27],1) ,MOV(16#c6e0_0bf3,Wrk[1]) MOV(16#3da8_8fc2,Wrk[0]) COP(Wrk[0],K[28],1) ,MOV(16#d5a7_9147,Wrk[1]) MOV(16#930a_a725,Wrk[0]) COP(Wrk[0],K[29],1) ,MOV(16#06ca_6351,Wrk[1]) MOV(16#e003_826f,Wrk[0]) COP(Wrk[0],K[30],1) ,MOV(16#1429_2967,Wrk[1]) MOV(16#0a0e_6e70,Wrk[0]) COP(Wrk[0],K[31],1) ,MOV(16#27b7_0a85,Wrk[1]) MOV(16#46d2_2ffc,Wrk[0]) COP(Wrk[0],K[32],1) ,MOV(16#2e1b_2138,Wrk[1]) MOV(16#5c26_c926,Wrk[0]) COP(Wrk[0],K[33],1) ,MOV(16#4d2c_6dfc,Wrk[1]) MOV(16#5ac4_2aed,Wrk[0]) COP(Wrk[0],K[34],1) ,MOV(16#5338_0d13,Wrk[1]) MOV(16#9d95_b3df,Wrk[0]) COP(Wrk[0],K[35],1) ,MOV(16#650a_7354,Wrk[1]) MOV(16#8baf_63de,Wrk[0]) COP(Wrk[0],K[36],1) ,MOV(16#766a_0abb,Wrk[1]) MOV(16#3c77_b2a8,Wrk[0]) COP(Wrk[0],K[37],1) ,MOV(16#81c2_c92e,Wrk[1]) MOV(16#47ed_aee6,Wrk[0]) COP(Wrk[0],K[38],1) ,MOV(16#9272_2c85,Wrk[1]) MOV(16#1482_353b,Wrk[0]) COP(Wrk[0],K[39],1) ];
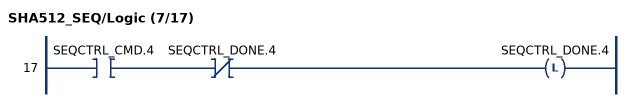
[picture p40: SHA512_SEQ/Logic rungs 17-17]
   17: XIC(SEQCTRL_CMD.4)XIO(SEQCTRL_DONE.4)OTL(SEQCTRL_DONE.4);
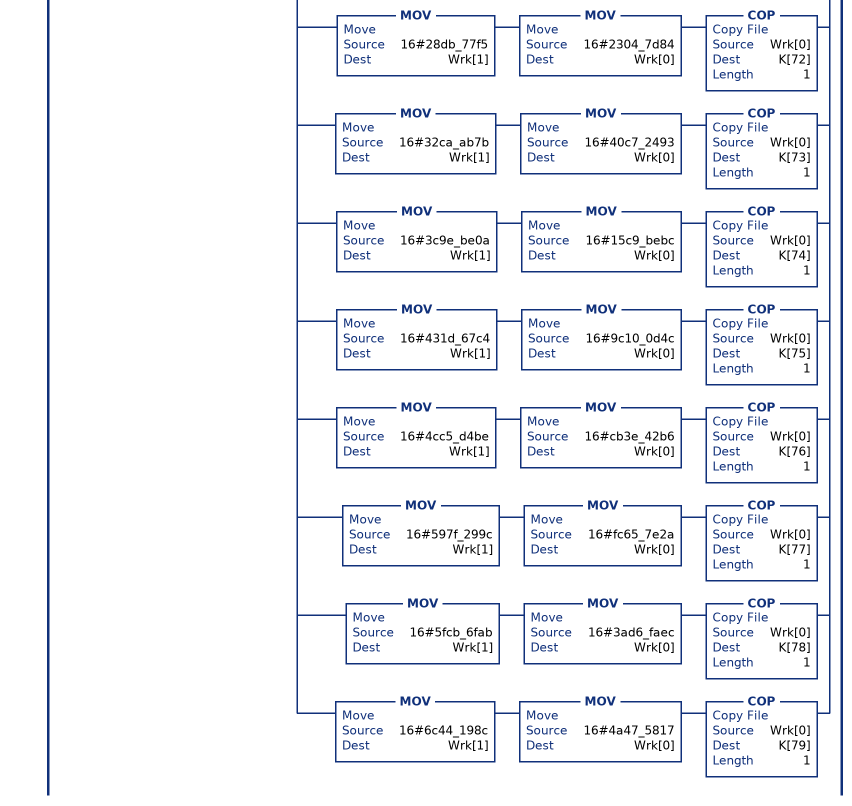
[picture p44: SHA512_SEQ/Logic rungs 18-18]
   // ===================================================
   // PART 5:  INITIALIZE K CONSTANTS - PART 2
   // ===================================================
   18: XIC(SEQCTRL_CMD.5)XIO(SEQCTRL_DONE.5)[MOV(16#a2bf_e8a1,Wrk[1]) MOV(16#4cf1_0364,Wrk[0]) COP(Wrk[0],K[40],1) ,MOV(16#a81a_664b,Wrk[1]) MOV(16#bc42_3001,Wrk[0]) COP(Wrk[0],K[41],1) ,MOV(16#c24b_8b70,Wrk[1]) MOV(16#d0f8_9791,Wrk[0]) COP(Wrk[0],K[42],1) ,MOV(16#c76c_51a3,Wrk[1]) MOV(16#0654_be30,Wrk[0]) COP(Wrk[0],K[43],1) ,MOV(16#d192_e819,Wrk[1]) MOV(16#d6ef_5218,Wrk[0]) COP(Wrk[0],K[44],1) ,MOV(16#d699_0624,Wrk[1]) MOV(16#5565_a910,Wrk[0]) COP(Wrk[0],K[45],1) ,MOV(16#f40e_3585,Wrk[1]) MOV(16#5771_202a,Wrk[0]) COP(Wrk[0],K[46],1) ,MOV(16#106a_a070,Wrk[1]) MOV(16#32bb_d1b8,Wrk[0]) COP(Wrk[0],K[47],1) ,MOV(16#19a4_c116,Wrk[1]) MOV(16#b8d2_d0c8,Wrk[0]) COP(Wrk[0],K[48],1) ,MOV(16#1e37_6c08,Wrk[1]) MOV(16#5141_ab53,Wrk[0]) COP(Wrk[0],K[49],1) ,MOV(16#2748_774c,Wrk[1]) MOV(16#df8e_eb99,Wrk[0]) COP(Wrk[0],K[50],1) ,MOV(16#34b0_bcb5,Wrk[1]) MOV(16#e19b_48a8,Wrk[0]) COP(Wrk[0],K[51],1) ,MOV(16#391c_0cb3,Wrk[1]) MOV(16#c5c9_5a63,Wrk[0]) COP(Wrk[0],K[52],1) ,MOV(16#4ed8_aa4a,Wrk[1]) MOV(16#e341_8acb,Wrk[0]) COP(Wrk[0],K[53],1) ,MOV(16#5b9c_ca4f,Wrk[1]) MOV(16#7763_e373,Wrk[0]) COP(Wrk[0],K[54],1) ,MOV(16#682e_6ff3,Wrk[1]) MOV(16#d6b2_b8a3,Wrk[0]) COP(Wrk[0],K[55],1) ,MOV(16#748f_82ee,Wrk[1]) MOV(16#5def_b2fc,Wrk[0]) COP(Wrk[0],K[56],1) ,MOV(16#78a5_636f,Wrk[1]) MOV(16#4317_2f60,Wrk[0]) COP(Wrk[0],K[57],1) ,MOV(16#84c8_7814,Wrk[1]) MOV(16#a1f0_ab72,Wrk[0]) COP(Wrk[0],K[58],1) ,MOV(16#8cc7_0208,Wrk[1]) MOV(16#1a64_39ec,Wrk[0]) COP(Wrk[0],K[59],1) ,MOV(16#90be_fffa,Wrk[1]) MOV(16#2363_1e28,Wrk[0]) COP(Wrk[0],K[60],1) ,MOV(16#a450_6ceb,Wrk[1]) MOV(16#de82_bde9,Wrk[0]) COP(Wrk[0],K[61],1) ,MOV(16#bef9_a3f7,Wrk[1]) MOV(16#b2c6_7915,Wrk[0]) COP(Wrk[0],K[62],1) ,MOV(16#c671_78f2,Wrk[1]) MOV(16#e372_532b,Wrk[0]) COP(Wrk[0],K[63],1) ,MOV(16#ca27_3ece,Wrk[1]) MOV(16#ea26_619c,Wrk[0]) COP(Wrk[0],K[64],1) ,MOV(16#d186_b8c7,Wrk[1]) MOV(16#21c0_c207,Wrk[0]) COP(Wrk[0],K[65],1) ,MOV(16#eada_7dd6,Wrk[1]) MOV(16#cde0_eb1e,Wrk[0]) COP(Wrk[0],K[66],1) ,MOV(16#f57d_4f7f,Wrk[1]) MOV(16#ee6e_d178,Wrk[0]) COP(Wrk[0],K[67],1) ,MOV(16#06f0_67aa,Wrk[1]) MOV(16#7217_6fba,Wrk[0]) COP(Wrk[0],K[68],1) ,MOV(16#0a63_7dc5,Wrk[1]) MOV(16#a2c8_98a6,Wrk[0]) COP(Wrk[0],K[69],1) ,MOV(16#113f_9804,Wrk[1]) MOV(16#bef9_0dae,Wrk[0]) COP(Wrk[0],K[70],1) ,MOV(16#1b71_0b35,Wrk[1]) MOV(16#131c_471b,Wrk[0]) COP(Wrk[0],K[71],1) ,MOV(16#28db_77f5,Wrk[1]) MOV(16#2304_7d84,Wrk[0]) COP(Wrk[0],K[72],1) ,MOV(16#32ca_ab7b,Wrk[1]) MOV(16#40c7_2493,Wrk[0]) COP(Wrk[0],K[73],1) ,MOV(16#3c9e_be0a,Wrk[1]) MOV(16#15c9_bebc,Wrk[0]) COP(Wrk[0],K[74],1) ,MOV(16#431d_67c4,Wrk[1]) MOV(16#9c10_0d4c,Wrk[0]) COP(Wrk[0],K[75],1) ,MOV(16#4cc5_d4be,Wrk[1]) MOV(16#cb3e_42b6,Wrk[0]) COP(Wrk[0],K[76],1) ,MOV(16#597f_299c,Wrk[1]) MOV(16#fc65_7e2a,Wrk[0]) COP(Wrk[0],K[77],1) ,MOV(16#5fcb_6fab,Wrk[1]) MOV(16#3ad6_faec,Wrk[0]) COP(Wrk[0],K[78],1) ,MOV(16#6c44_198c,Wrk[1]) MOV(16#4a47_5817,Wrk[0]) COP(Wrk[0],K[79],1) ];
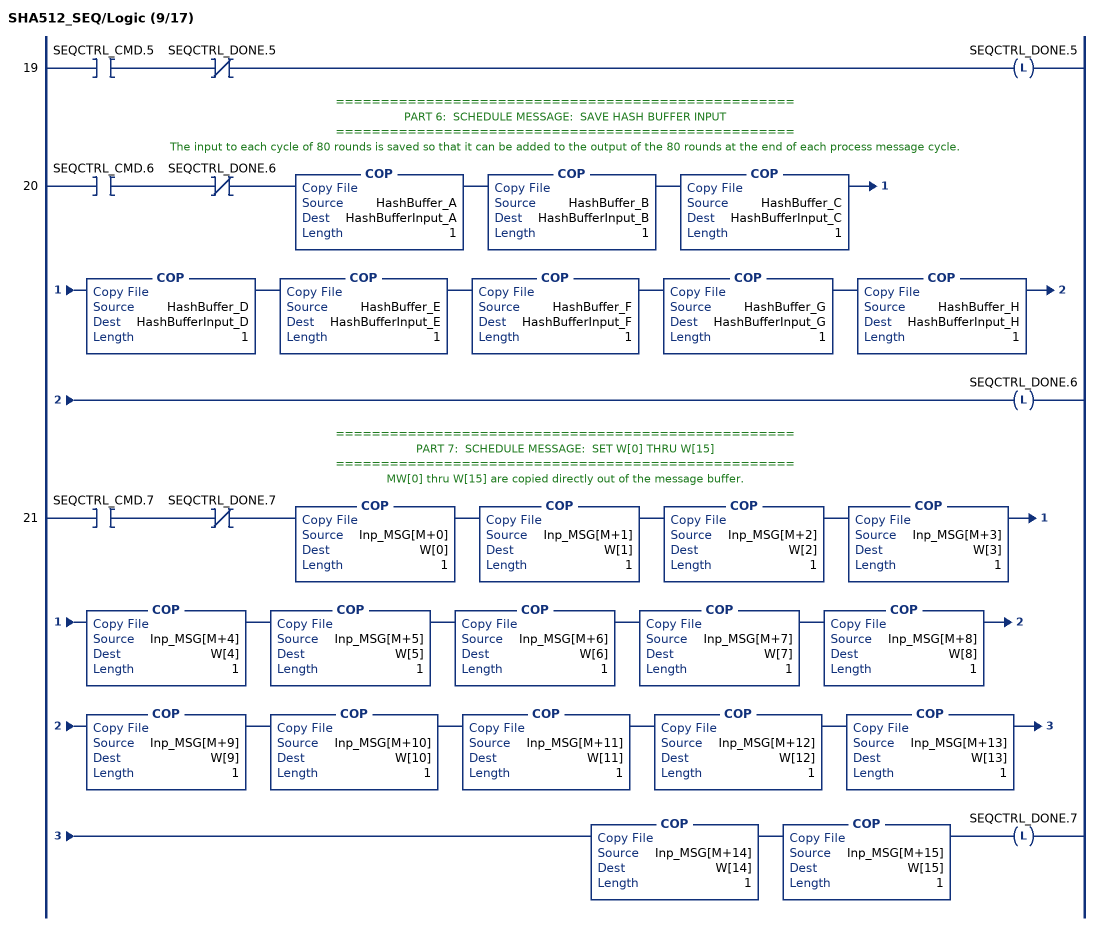
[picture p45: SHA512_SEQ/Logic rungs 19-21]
   19: XIC(SEQCTRL_CMD.5)XIO(SEQCTRL_DONE.5)OTL(SEQCTRL_DONE.5);
   // ===================================================
   // PART 6:  SCHEDULE MESSAGE:  SAVE HASH BUFFER INPUT
   // ===================================================
   // The input to each cycle of 80 rounds is saved so that it can be added to the output of the 80 rounds at the end of each process message cycle.
   20: XIC(SEQCTRL_CMD.6)XIO(SEQCTRL_DONE.6)COP(HashBuffer_A,HashBufferInput_A,1)COP(HashBuffer_B,HashBufferInput_B,1)COP(HashBuffer_C,HashBufferInput_C,1)COP(HashBuffer_D,HashBufferInput_D,1)COP(HashBuffer_E,HashBufferInput_E,1)COP(HashBuffer_F,HashBufferInput_F,1)COP(HashBuffer_G,HashBufferInput_G,1)COP(HashBuffer_H,HashBufferInput_H,1)OTL(SEQCTRL_DONE.6);
   // ===================================================
   // PART 7:  SCHEDULE MESSAGE:  SET W[0] THRU W[15]
   // ===================================================
   // MW[0] thru W[15] are copied directly out of the message buffer.
   21: XIC(SEQCTRL_CMD.7)XIO(SEQCTRL_DONE.7)COP(Inp_MSG[M+0],W[0],1)COP(Inp_MSG[M+1],W[1],1)COP(Inp_MSG[M+2],W[2],1)COP(Inp_MSG[M+3],W[3],1)COP(Inp_MSG[M+4],W[4],1)COP(Inp_MSG[M+5],W[5],1)COP(Inp_MSG[M+6],W[6],1)COP(Inp_MSG[M+7],W[7],1)COP(Inp_MSG[M+8],W[8],1)COP(Inp_MSG[M+9],W[9],1)COP(Inp_MSG[M+10],W[10],1)COP(Inp_MSG[M+11],W[11],1)COP(Inp_MSG[M+12],W[12],1)COP(Inp_MSG[M+13],W[13],1)COP(Inp_MSG[M+14],W[14],1)COP(Inp_MSG[M+15],W[15],1)OTL(SEQCTRL_DONE.7);
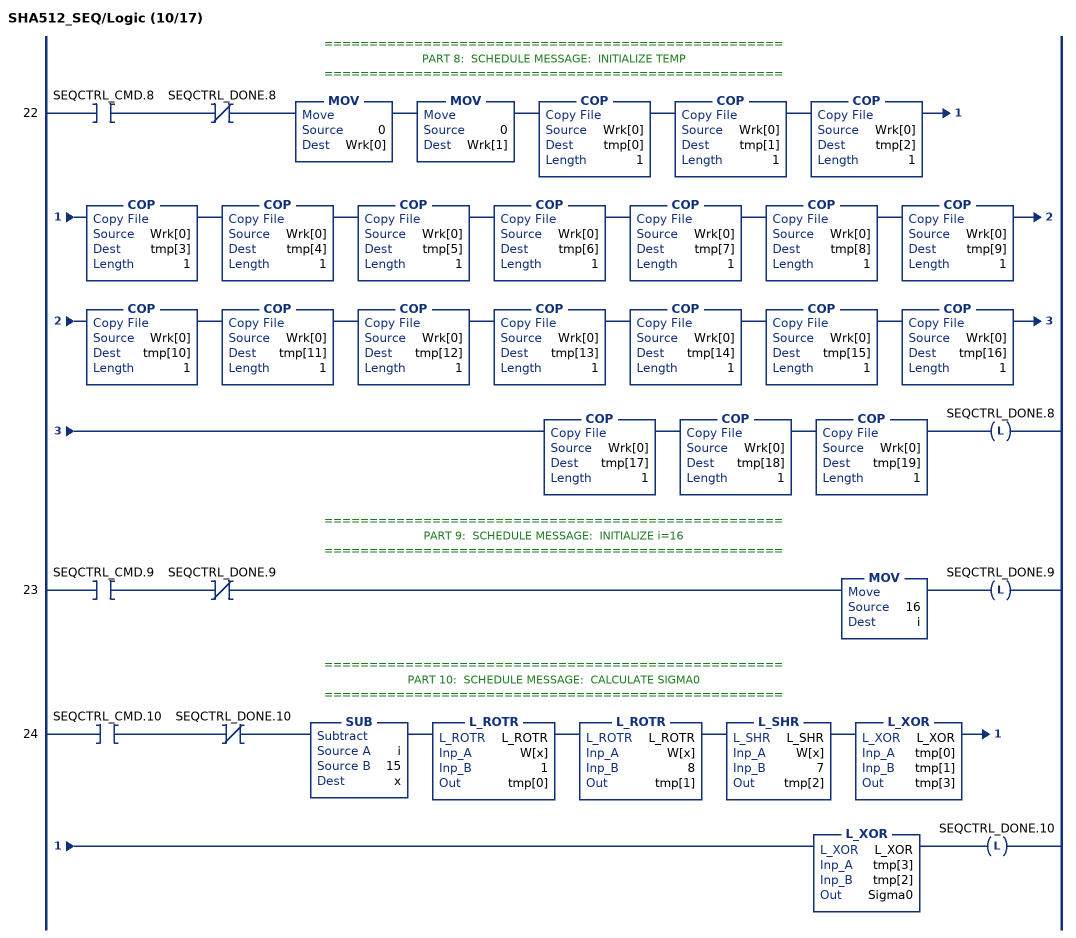
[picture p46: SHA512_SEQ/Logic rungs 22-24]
   // ===================================================
   // PART 8:  SCHEDULE MESSAGE:  INITIALIZE TEMP
   // ===================================================
   22: XIC(SEQCTRL_CMD.8)XIO(SEQCTRL_DONE.8)MOV(0,Wrk[0])MOV(0,Wrk[1])COP(Wrk[0],tmp[0],1)COP(Wrk[0],tmp[1],1)COP(Wrk[0],tmp[2],1)COP(Wrk[0],tmp[3],1)COP(Wrk[0],tmp[4],1)COP(Wrk[0],tmp[5],1)COP(Wrk[0],tmp[6],1)COP(Wrk[0],tmp[7],1)COP(Wrk[0],tmp[8],1)COP(Wrk[0],tmp[9],1)COP(Wrk[0],tmp[10],1)COP(Wrk[0],tmp[11],1)COP(Wrk[0],tmp[12],1)COP(Wrk[0],tmp[13],1)COP(Wrk[0],tmp[14],1)COP(Wrk[0],tmp[15],1)COP(Wrk[0],tmp[16],1)COP(Wrk[0],tmp[17],1)COP(Wrk[0],tmp[18],1)COP(Wrk[0],tmp[19],1)OTL(SEQCTRL_DONE.8);
   // ===================================================
   // PART 9:  SCHEDULE MESSAGE:  INITIALIZE i=16
   // ===================================================
   23: XIC(SEQCTRL_CMD.9)XIO(SEQCTRL_DONE.9)MOV(16,i)OTL(SEQCTRL_DONE.9);
   // ===================================================
   // PART 10:  SCHEDULE MESSAGE:  CALCULATE SIGMA0
   // ===================================================
   24: XIC(SEQCTRL_CMD.10)XIO(SEQCTRL_DONE.10)SUB(i,15,x)L_ROTR(L_ROTR,W[x],1,tmp[0])L_ROTR(L_ROTR,W[x],8,tmp[1])L_SHR(L_SHR,W[x],7,tmp[2])L_XOR(L_XOR,tmp[0],tmp[1],tmp[3])L_XOR(L_XOR,tmp[3],tmp[2],Sigma0)OTL(SEQCTRL_DONE.10);
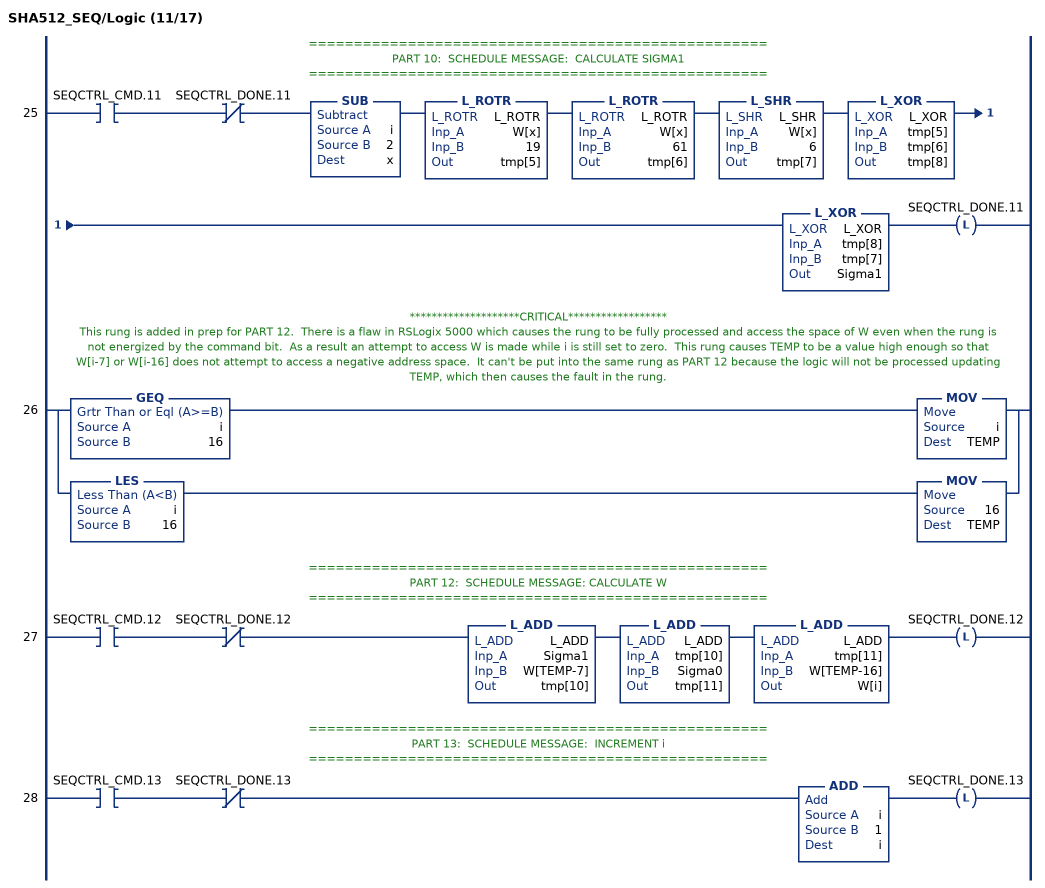
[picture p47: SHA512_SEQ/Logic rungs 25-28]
   // ===================================================
   // PART 10:  SCHEDULE MESSAGE:  CALCULATE SIGMA1
   // ===================================================
   25: XIC(SEQCTRL_CMD.11)XIO(SEQCTRL_DONE.11)SUB(i,2,x)L_ROTR(L_ROTR,W[x],19,tmp[5])L_ROTR(L_ROTR,W[x],61,tmp[6])L_SHR(L_SHR,W[x],6,tmp[7])L_XOR(L_XOR,tmp[5],tmp[6],tmp[8])L_XOR(L_XOR,tmp[8],tmp[7],Sigma1)OTL(SEQCTRL_DONE.11);
   // ********************CRITICAL******************
   // This rung is added in prep for PART 12.  There is a flaw in RSLogix 5000 which causes the rung to be fully processed and access the space of W even when the rung is not energized by the command bit.  As a result an attempt to access W is made while i is still set to zero.  This rung causes TEMP to be a value high enough so that W[i-7] or W[i-16] does not attempt to access a negative address space.  It can't be put into the same rung as PART 12 because the logic will not be processed updating TEMP, which then causes the fault in the rung.
   26: [GEQ(i,16) MOV(i,TEMP) ,LES(i,16) MOV(16,TEMP) ];
   // ===================================================
   // PART 12:  SCHEDULE MESSAGE: CALCULATE W
   // ===================================================
   27: XIC(SEQCTRL_CMD.12)XIO(SEQCTRL_DONE.12)L_ADD(L_ADD,Sigma1,W[TEMP-7],tmp[10])L_ADD(L_ADD,tmp[10],Sigma0,tmp[11])L_ADD(L_ADD,tmp[11],W[TEMP-16],W[i])OTL(SEQCTRL_DONE.12);
   // ===================================================
   // PART 13:  SCHEDULE MESSAGE:  INCREMENT i
   // ===================================================
   28: XIC(SEQCTRL_CMD.13)XIO(SEQCTRL_DONE.13)ADD(i,1,i)OTL(SEQCTRL_DONE.13);
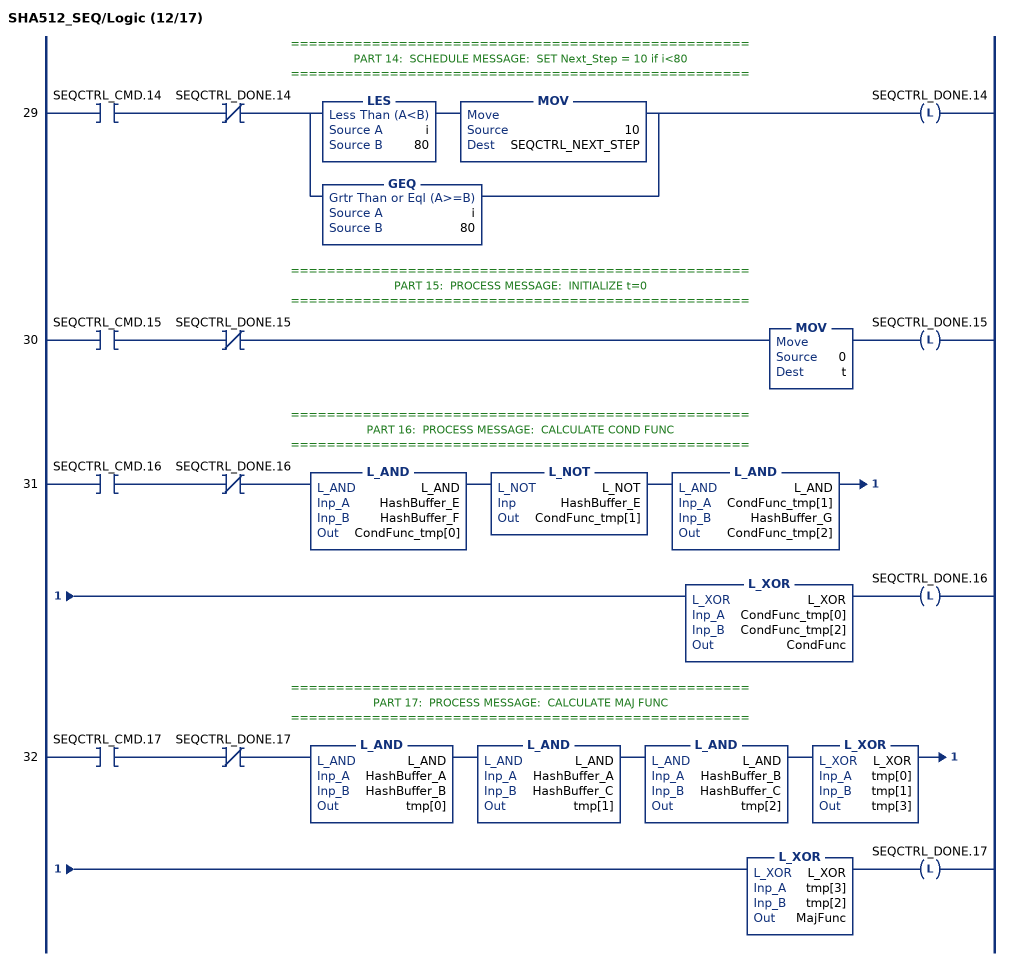
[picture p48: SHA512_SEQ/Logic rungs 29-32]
   // ===================================================
   // PART 14:  SCHEDULE MESSAGE:  SET Next_Step = 10 if i<80
   // ===================================================
   29: XIC(SEQCTRL_CMD.14)XIO(SEQCTRL_DONE.14)[LES(i,80) MOV(10,SEQCTRL_NEXT_STEP) ,GEQ(i,80) ]OTL(SEQCTRL_DONE.14);
   // ===================================================
   // PART 15:  PROCESS MESSAGE:  INITIALIZE t=0
   // ===================================================
   30: XIC(SEQCTRL_CMD.15)XIO(SEQCTRL_DONE.15)MOV(0,t)OTL(SEQCTRL_DONE.15);
   // ===================================================
   // PART 16:  PROCESS MESSAGE:  CALCULATE COND FUNC
   // ===================================================
   31: XIC(SEQCTRL_CMD.16)XIO(SEQCTRL_DONE.16)L_AND(L_AND,HashBuffer_E,HashBuffer_F,CondFunc_tmp[0])L_NOT(L_NOT,HashBuffer_E,CondFunc_tmp[1])L_AND(L_AND,CondFunc_tmp[1],HashBuffer_G,CondFunc_tmp[2])L_XOR(L_XOR,CondFunc_tmp[0],CondFunc_tmp[2],CondFunc)OTL(SEQCTRL_DONE.16);
   // ===================================================
   // PART 17:  PROCESS MESSAGE:  CALCULATE MAJ FUNC
   // ===================================================
   32: XIC(SEQCTRL_CMD.17)XIO(SEQCTRL_DONE.17)L_AND(L_AND,HashBuffer_A,HashBuffer_B,tmp[0])L_AND(L_AND,HashBuffer_A,HashBuffer_C,tmp[1])L_AND(L_AND,HashBuffer_B,HashBuffer_C,tmp[2])L_XOR(L_XOR,tmp[0],tmp[1],tmp[3])L_XOR(L_XOR,tmp[3],tmp[2],MajFunc)OTL(SEQCTRL_DONE.17);
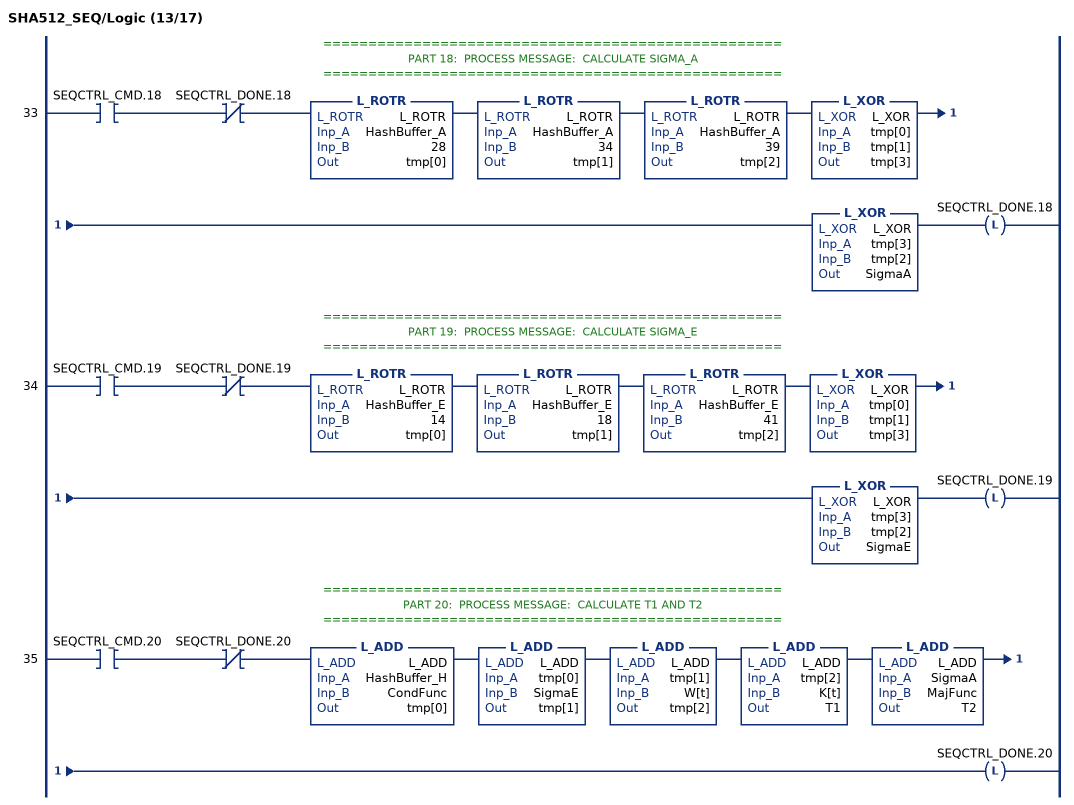
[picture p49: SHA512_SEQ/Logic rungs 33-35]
   // ===================================================
   // PART 18:  PROCESS MESSAGE:  CALCULATE SIGMA_A
   // ===================================================
   33: XIC(SEQCTRL_CMD.18)XIO(SEQCTRL_DONE.18)L_ROTR(L_ROTR,HashBuffer_A,28,tmp[0])L_ROTR(L_ROTR,HashBuffer_A,34,tmp[1])L_ROTR(L_ROTR,HashBuffer_A,39,tmp[2])L_XOR(L_XOR,tmp[0],tmp[1],tmp[3])L_XOR(L_XOR,tmp[3],tmp[2],SigmaA)OTL(SEQCTRL_DONE.18);
   // ===================================================
   // PART 19:  PROCESS MESSAGE:  CALCULATE SIGMA_E
   // ===================================================
   34: XIC(SEQCTRL_CMD.19)XIO(SEQCTRL_DONE.19)L_ROTR(L_ROTR,HashBuffer_E,14,tmp[0])L_ROTR(L_ROTR,HashBuffer_E,18,tmp[1])L_ROTR(L_ROTR,HashBuffer_E,41,tmp[2])L_XOR(L_XOR,tmp[0],tmp[1],tmp[3])L_XOR(L_XOR,tmp[3],tmp[2],SigmaE)OTL(SEQCTRL_DONE.19);
   // ===================================================
   // PART 20:  PROCESS MESSAGE:  CALCULATE T1 AND T2
   // ===================================================
   35: XIC(SEQCTRL_CMD.20)XIO(SEQCTRL_DONE.20)L_ADD(L_ADD,HashBuffer_H,CondFunc,tmp[0])L_ADD(L_ADD,tmp[0],SigmaE,tmp[1])L_ADD(L_ADD,tmp[1],W[t],tmp[2])L_ADD(L_ADD,tmp[2],K[t],T1)L_ADD(L_ADD,SigmaA,MajFunc,T2)OTL(SEQCTRL_DONE.20);
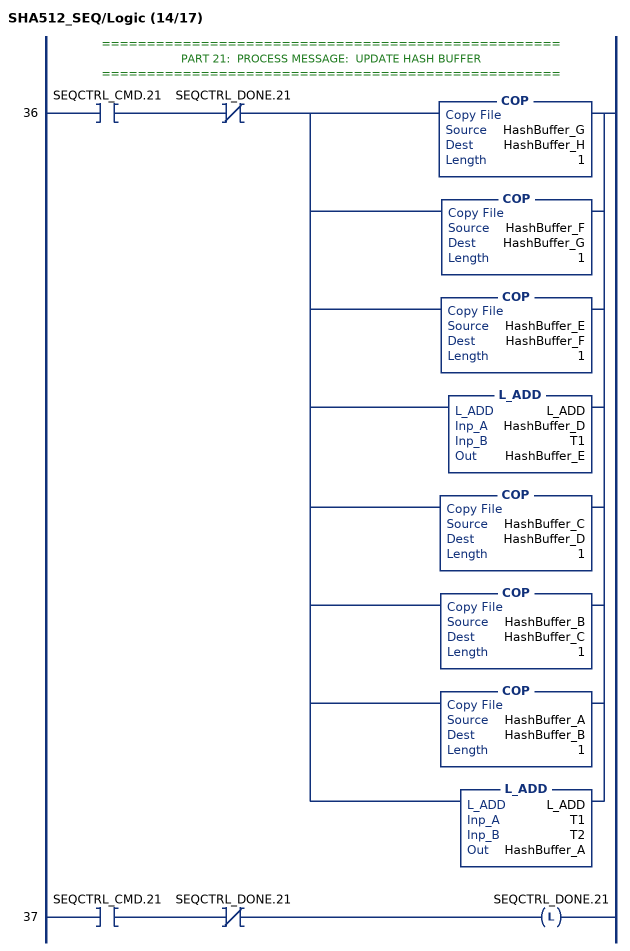
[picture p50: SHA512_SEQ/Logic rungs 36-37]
   // ===================================================
   // PART 21:  PROCESS MESSAGE:  UPDATE HASH BUFFER
   // ===================================================
   36: XIC(SEQCTRL_CMD.21)XIO(SEQCTRL_DONE.21)[COP(HashBuffer_G,HashBuffer_H,1) ,COP(HashBuffer_F,HashBuffer_G,1) ,COP(HashBuffer_E,HashBuffer_F,1) ,L_ADD(L_ADD,HashBuffer_D,T1,HashBuffer_E) ,COP(HashBuffer_C,HashBuffer_D,1) ,COP(HashBuffer_B,HashBuffer_C,1) ,COP(HashBuffer_A,HashBuffer_B,1) ,L_ADD(L_ADD,T1,T2,HashBuffer_A) ];
   37: XIC(SEQCTRL_CMD.21)XIO(SEQCTRL_DONE.21)OTL(SEQCTRL_DONE.21);
